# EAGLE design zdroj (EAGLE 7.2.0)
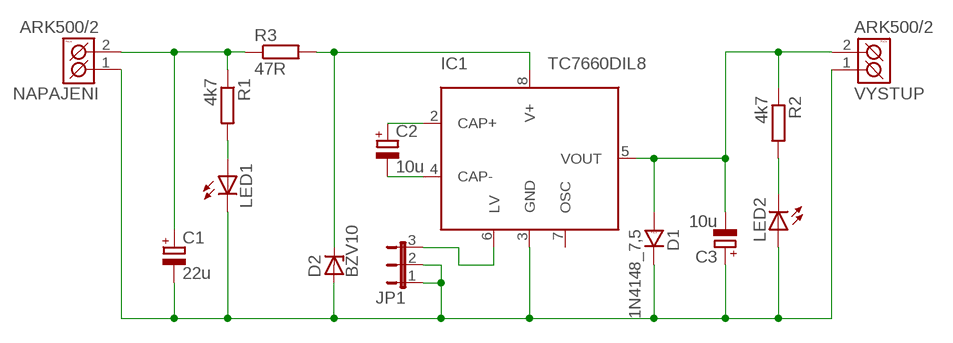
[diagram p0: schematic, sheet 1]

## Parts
C1  22u  CPOL-EUE22-6AXIAL  [E22-6]
C2  10u  CPOL-EUE22-6AXIAL  [E22-6]
C3  10u  CPOL-EUE22-6AXIAL  [E22-6]
D1  1N4148_7,5  [D-7,5]
D2  BZV10  [DO34Z7]
IC1  TC7660DIL8  [DIL8]
JP1  JP2E  [JP2]
LED1  LED3MM  [LED3MM]
LED2  LED3MM  [LED3MM]
NAPAJENI  ARK500/2  [ARK500/2]
R1  4k7  R-EU_0207/10  [0207/10]
R2  4k7  R-EU_0207/10  [0207/10]
R3  47R  R-EU_0207/10  [0207/10]
VYSTUP  ARK500/2  [ARK500/2]

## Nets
N$1: LED1.A R1.2
N$2: C1.+ NAPAJENI.2(K2) R1.1 R3.1
N$3: D2.C IC1.8(V+) R3.2
N$4: C1.- C3.+ D1.K D2.A IC1.3(GND) JP1.1 JP1.2 LED1.K(C) LED2.A NAPAJENI.1(K1) VYSTUP.1(K1)
N$5: C2.- IC1.4(CAP-)
N$6: LED2.K(C) R2.2
N$7: C3.- D1.A IC1.5(VOUT) R2.1 VYSTUP.2(K2)
N$8: C2.+ IC1.2(CAP+)
N$9: IC1.6(LV) JP1.3
Unconnected: IC1.7(OSC)

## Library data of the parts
C1-C3 = rcl:CPOL-EU: POLARIZED CAPACITOR, European symbol
D1 = #PaJa_21:1N4148: Univerzalni dioda - 0,15A, 75V
D2 = diode:BZV10: Z DIODE
IC1 = microchip_tc7660:TC7660: TC7660 Charge Pump DC-to-DC Voltage Converter
JP1 = jumper:JP2E: JUMPER
LED1 LED2 = led:LED: LED
NAPAJENI VYSTUP = #PaJa_21:ARK500/2: Svorkovnice - roztec 5mm - dvojita
R1-R3 = rcl:R-EU_: RESISTOR, European symbol

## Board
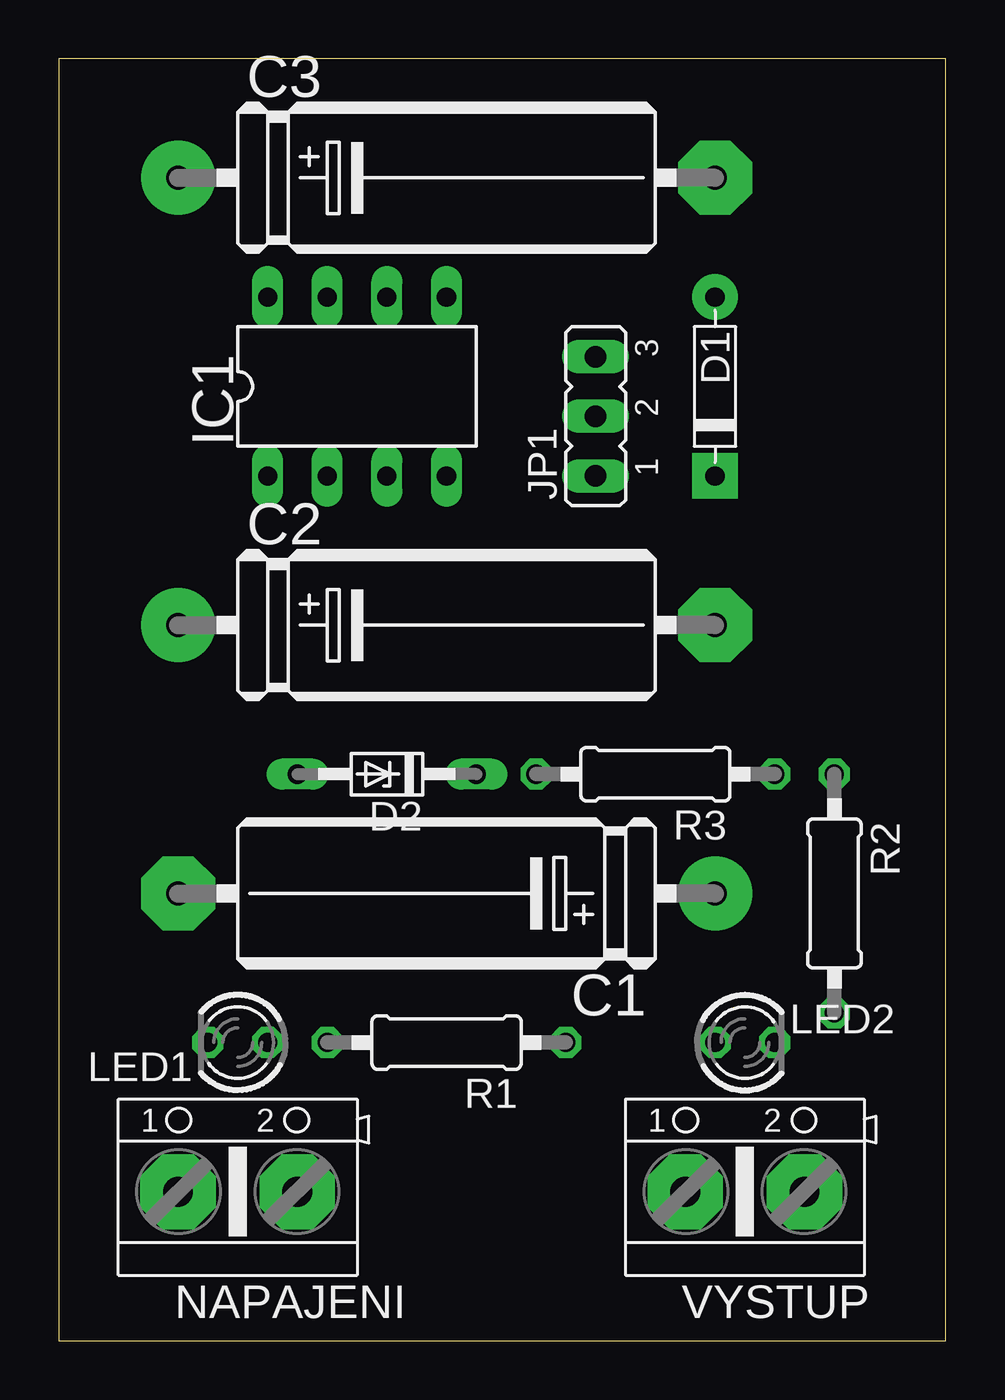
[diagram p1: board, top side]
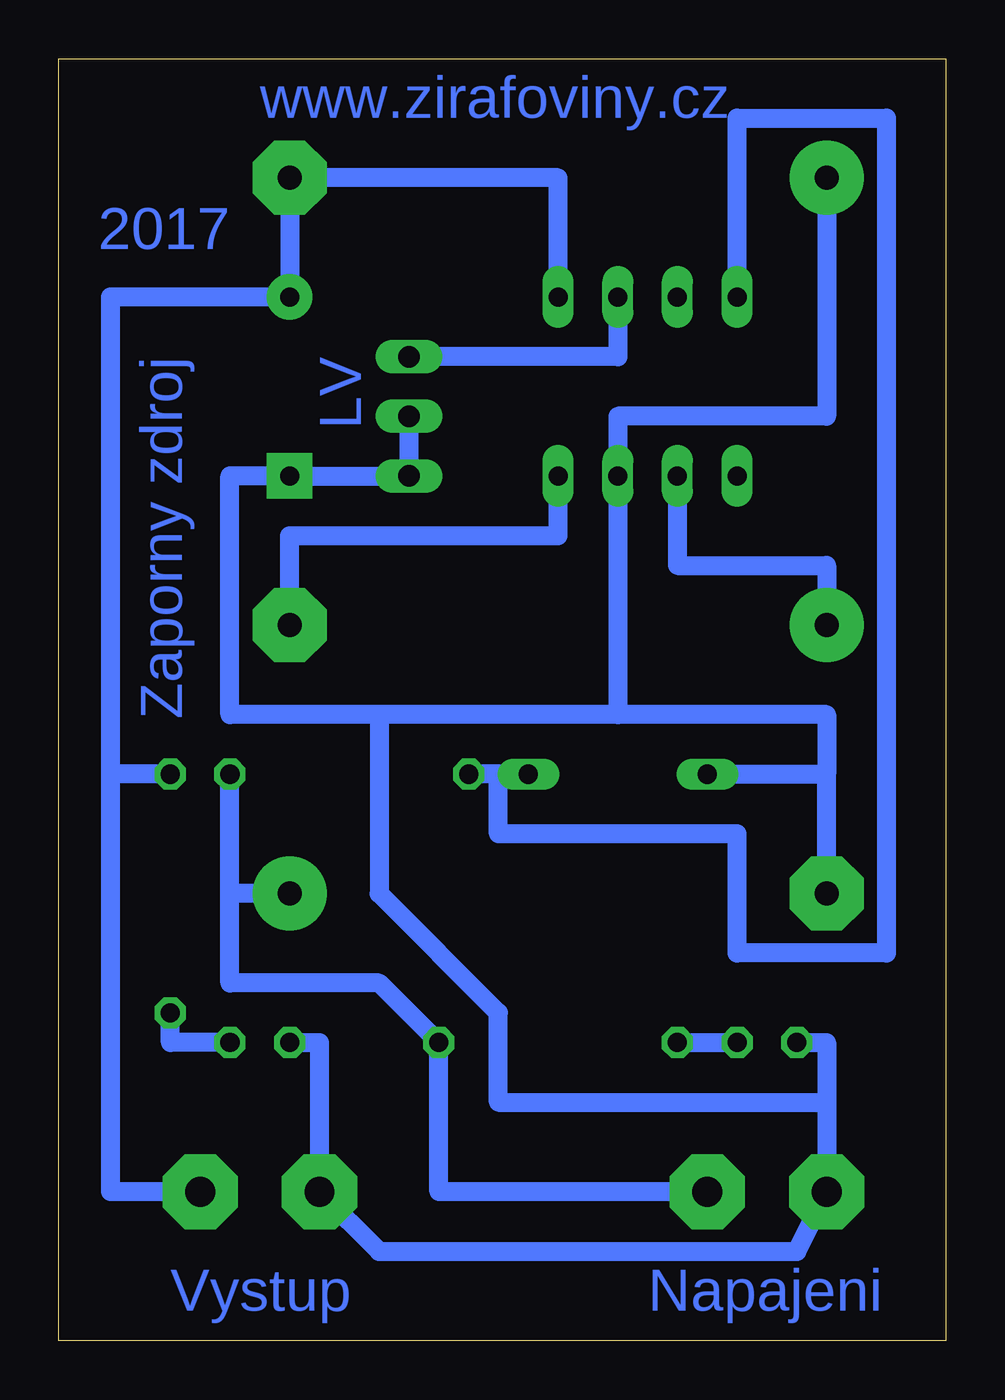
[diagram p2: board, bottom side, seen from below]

Size 37.77 x 54.6 mm. Coordinates in mm from the lower left corner, seen from the top.
Outline: 0,0 37.77,0 37.77,54.6 0,54.6 0,0
Copper layers (1*16): Top 0.035mm / dielectric 1.5mm / Bottom 0.035mm
Design rules "default": minimum track width 10mil, minimum drill 24mil, track to track 8mil, track to pad 8mil, pad to pad 8mil, via to via 8mil, smd to smd 8mil, copper to edge 40mil, drill to drill 8mil, minimum pad ring 10mil, minimum via ring 8mil, stop-mask expansion 4mil, vias tented up to drill 0mil, thermal gap 10mil

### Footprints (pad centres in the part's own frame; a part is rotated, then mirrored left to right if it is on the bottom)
E22-6 = drill 1.016 pad 3.15: + -11.43,0 | drill 1.016 pad 3.15 octagon: - 11.43,0
D-7,5 = drill 0.813 pad 1.93: A -3.81,0 | drill 0.813 pad 1.93 square: K 3.81,0
DO34Z7 = drill 0.813 long: A 3.81,0; C -3.81,0
DIL8 = drill 0.813 long: 1 -3.81,-3.81; 2 -1.27,-3.81; 3 1.27,-3.81; 4 3.81,-3.81; 5 3.81,3.81; 6 1.27,3.81; 7 -1.27,3.81; 8 -3.81,3.81
JP2 = drill 0.914 long: 1 -2.54,0; 2 0,0; 3 2.54,0
LED3MM = drill 0.813 octagon: A -1.27,0; K 1.27,0
ARK500/2 = drill 1.27 pad 3.2 octagon: 1 -2.54,0; 2 2.54,0
0207/10 = drill 0.813 octagon: 1 -5.08,0; 2 5.08,0

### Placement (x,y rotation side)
C1  16.51,19.05 180 top
C2  16.51,30.48 0 top
C3  16.51,49.53 0 top
D1  27.94,40.64 270 top
D2  13.97,24.13 180 top
IC1  12.7,40.64 0 top
JP1  22.86,39.37 90 top
LED1  7.62,12.7 180 top
LED2  29.21,12.7 0 top
NAPAJENI  7.62,6.35 0 top
R1  16.51,12.7 180 top
R2  33.02,19.05 270 top
R3  25.4,24.13 180 top
VYSTUP  29.21,6.35 0 top

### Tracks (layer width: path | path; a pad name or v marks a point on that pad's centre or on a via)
N$1
  Bottom 0.813: R1.2 LED1.A
N$2
  Bottom 0.813: NAPAJENI.2 21.59,6.35 R1.1 24.13,15.24 30.48,15.24 30.48,19.05 | C1.+ 30.48,19.05 | 30.48,19.05 R3.1
N$3
  Bottom 0.813: D2.C 19.05,24.13 | 19.05,24.13 R3.2 | IC1.8 8.89,52.07 2.54,52.07 2.54,16.51 8.89,16.51 8.89,21.59 19.05,21.59 19.05,24.13
N$4
  Bottom 0.813: D2.A 5.08,24.13 | 5.08,24.13 5.08,26.67 13.97,26.67 | 13.97,26.67 IC1.3 13.97,39.37 5.08,39.37 C3.+ | C1.- 5.08,24.13 | 13.97,26.67 24.13,26.67 | 24.13,26.67 24.13,19.05 19.05,13.97 19.05,10.16 5.08,10.16 | 24.13,26.67 30.48,26.67 30.48,36.83 D1.K JP1.1 JP1.2 | 5.08,10.16 5.08,12.7 LED1.K | 5.08,10.16 NAPAJENI.1 6.35,3.81 24.13,3.81 VYSTUP.1 26.67,12.7 LED2.A
N$5
  Bottom 0.813: C2.- 27.94,34.29 16.51,34.29 IC1.4
N$6
  Bottom 0.813: LED2.K 33.02,12.7 R2.2
N$7
  Bottom 0.813: IC1.5 16.51,49.53 C3.- D1.A 35.56,44.45 35.56,24.13 | VYSTUP.2 35.56,6.35 35.56,24.13 | R2.1 35.56,24.13
N$8
  Bottom 0.813: IC1.2 11.43,33.02 5.08,33.02 C2.+
N$9
  Bottom 0.813: IC1.6 13.97,41.91 JP1.3

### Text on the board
Bottom: www.zirafoviny.cz | 2017 | LV | Zaporny zdroj | Napajeni | Vystup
